ORGANIZATION_BLOCK OB 1
BEGIN
	// Check ANY pointer parameters
	CALL		FC 1 (
		FCANY1		:= P#M 10.0 BYTE 7,
		FCANY2		:= P#M 11.1 BOOL 13,
		FCANY3		:= M 12.2,
		FCANY4		:= P#DB50.DBX 10.0 DWORD 8,
		FCANY5		:= DB50.DBD 10,
		FCANY6		:= P#DBX 20.2 WORD 7,
		FCANY7		:= DB100.DBVAR2[2].V2,
		FCANY8		:= P#DB100.DBVAR2[2].V2, // awlsim extension
		FCANY9		:= P#DB100.DBVAR3, // awlsim extension
		FCANY10		:= P#DB100.DBVAR4, // awlsim extension
	)
	CALL		FB 1, DB 1 (
		FBANY1		:= P#M 10.0 BYTE 7,
		FBANY2		:= P#M 11.1 BOOL 13,
		FBANY3		:= M 12.2,
		FBANY4		:= P#DB50.DBX 10.0 DWORD 8,
		FBANY5		:= DB50.DBD 10,
		FBANY6		:= P#DBX 20.2 WORD 7,
		FBANY7		:= DB100.DBVAR2[2].V2,
		FBANY8		:= P#DB100.DBVAR2[2].V2, // awlsim extension
		FBANY9		:= P#DB100.DBVAR3, // awlsim extension
		FBANY10		:= P#DB100.DBVAR4, // awlsim extension
	)


	CALL SFC 46 // STOP CPU
END_ORGANIZATION_BLOCK


DATA_BLOCK DB 100
	STRUCT
		DBVAR1		: INT;
		DBVAR2		: ARRAY[1 .. 6] of STRUCT
			V1	: INT;
			V2	: INT;
		END_STRUCT;
		DBVAR3		: ARRAY[1 .. 4] of STRUCT
			A1	: INT;
		END_STRUCT
		DBVAR4		: ARRAY[1 .. 8] of BYTE;
	END_STRUCT;
BEGIN
END_DATA_BLOCK


FUNCTION FC 1 : VOID
	VAR_INPUT
		FCANY1		: ANY;
		FCANY2		: ANY;
		FCANY3		: ANY;
		FCANY4		: ANY;
		FCANY5		: ANY;
		FCANY6		: ANY;
		FCANY7		: ANY;
		FCANY8		: ANY;
		FCANY9		: ANY;
		FCANY10		: ANY;
	END_VAR
BEGIN
	L		P##FCANY1
	LAR1
	UD		DW#16#FF000000
	__ASSERT==	__ACCU 1,	DW#16#87000000
	L		B [AR1, P#0.0]
	__ASSERT==	__ACCU 1,	B#16#10	// S7
	L		B [AR1, P#1.0]
	__ASSERT==	__ACCU 1,	B#16#02	// BYTE
	L		W [AR1, P#2.0]
	__ASSERT==	__ACCU 1,	7	// count
	L		W [AR1, P#4.0]
	__ASSERT==	__ACCU 1,	0	// DB
	L		D [AR1, P#6.0]
	__ASSERT==	__ACCU 1,	P#M 10.0

	L		P##FCANY2
	LAR1
	UD		DW#16#FF000000
	__ASSERT==	__ACCU 1,	DW#16#87000000
	L		B [AR1, P#0.0]
	__ASSERT==	__ACCU 1,	B#16#10	// S7
	L		B [AR1, P#1.0]
	__ASSERT==	__ACCU 1,	B#16#01	// BOOL
	L		W [AR1, P#2.0]
	__ASSERT==	__ACCU 1,	13	// count
	L		W [AR1, P#4.0]
	__ASSERT==	__ACCU 1,	0	// DB
	L		D [AR1, P#6.0]
	__ASSERT==	__ACCU 1,	P#M 11.1

	L		P##FCANY3
	LAR1
	UD		DW#16#FF000000
	__ASSERT==	__ACCU 1,	DW#16#87000000
	L		B [AR1, P#0.0]
	__ASSERT==	__ACCU 1,	B#16#10	// S7
	L		B [AR1, P#1.0]
	__ASSERT==	__ACCU 1,	B#16#01	// BOOL
	L		W [AR1, P#2.0]
	__ASSERT==	__ACCU 1,	1	// count
	L		W [AR1, P#4.0]
	__ASSERT==	__ACCU 1,	0	// DB
	L		D [AR1, P#6.0]
	__ASSERT==	__ACCU 1,	P#M 12.2

	L		P##FCANY4
	LAR1
	UD		DW#16#FF000000
	__ASSERT==	__ACCU 1,	DW#16#87000000
	L		B [AR1, P#0.0]
	__ASSERT==	__ACCU 1,	B#16#10	// S7
	L		B [AR1, P#1.0]
	__ASSERT==	__ACCU 1,	B#16#06	// DWORD
	L		W [AR1, P#2.0]
	__ASSERT==	__ACCU 1,	8	// count
	L		W [AR1, P#4.0]
	__ASSERT==	__ACCU 1,	50	// DB
	L		D [AR1, P#6.0]
	__ASSERT==	__ACCU 1,	P#DBX 10.0

	L		P##FCANY5
	LAR1
	UD		DW#16#FF000000
	__ASSERT==	__ACCU 1,	DW#16#87000000
	L		B [AR1, P#0.0]
	__ASSERT==	__ACCU 1,	B#16#10	// S7
	L		B [AR1, P#1.0]
	__ASSERT==	__ACCU 1,	B#16#06	// DWORD
	L		W [AR1, P#2.0]
	__ASSERT==	__ACCU 1,	1	// count
	L		W [AR1, P#4.0]
	__ASSERT==	__ACCU 1,	50	// DB
	L		D [AR1, P#6.0]
	__ASSERT==	__ACCU 1,	P#DBX 10.0

	L		P##FCANY6
	LAR1
	UD		DW#16#FF000000
	__ASSERT==	__ACCU 1,	DW#16#87000000
	L		B [AR1, P#0.0]
	__ASSERT==	__ACCU 1,	B#16#10	// S7
	L		B [AR1, P#1.0]
	__ASSERT==	__ACCU 1,	B#16#04	// WORD
	L		W [AR1, P#2.0]
	__ASSERT==	__ACCU 1,	7	// count
	L		W [AR1, P#4.0]
	__ASSERT==	__ACCU 1,	0	// DB
	L		D [AR1, P#6.0]
	__ASSERT==	__ACCU 1,	P#DBX 20.2

	L		P##FCANY7
	LAR1
	UD		DW#16#FF000000
	__ASSERT==	__ACCU 1,	DW#16#87000000
	L		B [AR1, P#0.0]
	__ASSERT==	__ACCU 1,	B#16#10	// S7
	L		B [AR1, P#1.0]
	__ASSERT==	__ACCU 1,	B#16#05	// INT
	L		W [AR1, P#2.0]
	__ASSERT==	__ACCU 1,	1	// count
	L		W [AR1, P#4.0]
	__ASSERT==	__ACCU 1,	100	// DB
	L		D [AR1, P#6.0]
	__ASSERT==	__ACCU 1,	P#DBX 8.0

	L		P##FCANY8
	LAR1
	UD		DW#16#FF000000
	__ASSERT==	__ACCU 1,	DW#16#87000000
	L		B [AR1, P#0.0]
	__ASSERT==	__ACCU 1,	B#16#10	// S7
	L		B [AR1, P#1.0]
	__ASSERT==	__ACCU 1,	B#16#05	// INT
	L		W [AR1, P#2.0]
	__ASSERT==	__ACCU 1,	1	// count
	L		W [AR1, P#4.0]
	__ASSERT==	__ACCU 1,	100	// DB
	L		D [AR1, P#6.0]
	__ASSERT==	__ACCU 1,	P#DBX 8.0

	L		P##FCANY9
	LAR1
	UD		DW#16#FF000000
	__ASSERT==	__ACCU 1,	DW#16#87000000
	L		B [AR1, P#0.0]
	__ASSERT==	__ACCU 1,	B#16#10	// S7
	L		B [AR1, P#1.0]
	__ASSERT==	__ACCU 1,	B#16#06	// DWORD
	L		W [AR1, P#2.0]
	__ASSERT==	__ACCU 1,	2	// count
	L		W [AR1, P#4.0]
	__ASSERT==	__ACCU 1,	100	// DB
	L		D [AR1, P#6.0]
	__ASSERT==	__ACCU 1,	P#DBX 26.0

	L		P##FCANY10
	LAR1
	UD		DW#16#FF000000
	__ASSERT==	__ACCU 1,	DW#16#87000000
	L		B [AR1, P#0.0]
	__ASSERT==	__ACCU 1,	B#16#10	// S7
	L		B [AR1, P#1.0]
	__ASSERT==	__ACCU 1,	B#16#02	// BYTE
	L		W [AR1, P#2.0]
	__ASSERT==	__ACCU 1,	8	// count
	L		W [AR1, P#4.0]
	__ASSERT==	__ACCU 1,	100	// DB
	L		D [AR1, P#6.0]
	__ASSERT==	__ACCU 1,	P#DBX 34.0
END_FUNCTION


FUNCTION_BLOCK FB 1
	VAR_INPUT
		FBANY1		: ANY;
		FBANY2		: ANY;
		FBANY3		: ANY;
		FBANY4		: ANY;
		FBANY5		: ANY;
		FBANY6		: ANY;
		FBANY7		: ANY;
		FBANY8		: ANY;
		FBANY9		: ANY;
		FBANY10		: ANY;
	END_VAR
BEGIN
	L		P##FBANY1
	LAR1
	UD		DW#16#FF000000
	__ASSERT==	__ACCU 1,	DW#16#85000000
	L		B [AR1, P#0.0]
	__ASSERT==	__ACCU 1,	B#16#10	// S7
	L		B [AR1, P#1.0]
	__ASSERT==	__ACCU 1,	B#16#02	// BYTE
	L		W [AR1, P#2.0]
	__ASSERT==	__ACCU 1,	7	// count
	L		W [AR1, P#4.0]
	__ASSERT==	__ACCU 1,	0	// DB
	L		D [AR1, P#6.0]
	__ASSERT==	__ACCU 1,	P#M 10.0

	L		P##FBANY2
	LAR1
	UD		DW#16#FF000000
	__ASSERT==	__ACCU 1,	DW#16#85000000
	L		B [AR1, P#0.0]
	__ASSERT==	__ACCU 1,	B#16#10	// S7
	L		B [AR1, P#1.0]
	__ASSERT==	__ACCU 1,	B#16#01	// BOOL
	L		W [AR1, P#2.0]
	__ASSERT==	__ACCU 1,	13	// count
	L		W [AR1, P#4.0]
	__ASSERT==	__ACCU 1,	0	// DB
	L		D [AR1, P#6.0]
	__ASSERT==	__ACCU 1,	P#M 11.1

	L		P##FBANY3
	LAR1
	UD		DW#16#FF000000
	__ASSERT==	__ACCU 1,	DW#16#85000000
	L		B [AR1, P#0.0]
	__ASSERT==	__ACCU 1,	B#16#10	// S7
	L		B [AR1, P#1.0]
	__ASSERT==	__ACCU 1,	B#16#01	// BOOL
	L		W [AR1, P#2.0]
	__ASSERT==	__ACCU 1,	1	// count
	L		W [AR1, P#4.0]
	__ASSERT==	__ACCU 1,	0	// DB
	L		D [AR1, P#6.0]
	__ASSERT==	__ACCU 1,	P#M 12.2

	L		P##FBANY4
	LAR1
	UD		DW#16#FF000000
	__ASSERT==	__ACCU 1,	DW#16#85000000
	L		B [AR1, P#0.0]
	__ASSERT==	__ACCU 1,	B#16#10	// S7
	L		B [AR1, P#1.0]
	__ASSERT==	__ACCU 1,	B#16#06	// DWORD
	L		W [AR1, P#2.0]
	__ASSERT==	__ACCU 1,	8	// count
	L		W [AR1, P#4.0]
	__ASSERT==	__ACCU 1,	50	// DB
	L		D [AR1, P#6.0]
	__ASSERT==	__ACCU 1,	P#DBX 10.0

	L		P##FBANY5
	LAR1
	UD		DW#16#FF000000
	__ASSERT==	__ACCU 1,	DW#16#85000000
	L		B [AR1, P#0.0]
	__ASSERT==	__ACCU 1,	B#16#10	// S7
	L		B [AR1, P#1.0]
	__ASSERT==	__ACCU 1,	B#16#06	// DWORD
	L		W [AR1, P#2.0]
	__ASSERT==	__ACCU 1,	1	// count
	L		W [AR1, P#4.0]
	__ASSERT==	__ACCU 1,	50	// DB
	L		D [AR1, P#6.0]
	__ASSERT==	__ACCU 1,	P#DBX 10.0

	L		P##FBANY6
	LAR1
	UD		DW#16#FF000000
	__ASSERT==	__ACCU 1,	DW#16#85000000
	L		B [AR1, P#0.0]
	__ASSERT==	__ACCU 1,	B#16#10	// S7
	L		B [AR1, P#1.0]
	__ASSERT==	__ACCU 1,	B#16#04	// WORD
	L		W [AR1, P#2.0]
	__ASSERT==	__ACCU 1,	7	// count
	L		W [AR1, P#4.0]
	__ASSERT==	__ACCU 1,	0	// DB
	L		D [AR1, P#6.0]
	__ASSERT==	__ACCU 1,	P#DBX 20.2

	L		P##FBANY7
	LAR1
	UD		DW#16#FF000000
	__ASSERT==	__ACCU 1,	DW#16#85000000
	L		B [AR1, P#0.0]
	__ASSERT==	__ACCU 1,	B#16#10	// S7
	L		B [AR1, P#1.0]
	__ASSERT==	__ACCU 1,	B#16#05	// INT
	L		W [AR1, P#2.0]
	__ASSERT==	__ACCU 1,	1	// count
	L		W [AR1, P#4.0]
	__ASSERT==	__ACCU 1,	100	// DB
	L		D [AR1, P#6.0]
	__ASSERT==	__ACCU 1,	P#DBX 8.0

	L		P##FBANY8
	LAR1
	UD		DW#16#FF000000
	__ASSERT==	__ACCU 1,	DW#16#85000000
	L		B [AR1, P#0.0]
	__ASSERT==	__ACCU 1,	B#16#10	// S7
	L		B [AR1, P#1.0]
	__ASSERT==	__ACCU 1,	B#16#05	// INT
	L		W [AR1, P#2.0]
	__ASSERT==	__ACCU 1,	1	// count
	L		W [AR1, P#4.0]
	__ASSERT==	__ACCU 1,	100	// DB
	L		D [AR1, P#6.0]
	__ASSERT==	__ACCU 1,	P#DBX 8.0

	L		P##FBANY9
	LAR1
	UD		DW#16#FF000000
	__ASSERT==	__ACCU 1,	DW#16#85000000
	L		B [AR1, P#0.0]
	__ASSERT==	__ACCU 1,	B#16#10	// S7
	L		B [AR1, P#1.0]
	__ASSERT==	__ACCU 1,	B#16#06	// DWORD
	L		W [AR1, P#2.0]
	__ASSERT==	__ACCU 1,	2	// count
	L		W [AR1, P#4.0]
	__ASSERT==	__ACCU 1,	100	// DB
	L		D [AR1, P#6.0]
	__ASSERT==	__ACCU 1,	P#DBX 26.0

	L		P##FBANY10
	LAR1
	UD		DW#16#FF000000
	__ASSERT==	__ACCU 1,	DW#16#85000000
	L		B [AR1, P#0.0]
	__ASSERT==	__ACCU 1,	B#16#10	// S7
	L		B [AR1, P#1.0]
	__ASSERT==	__ACCU 1,	B#16#02	// BYTE
	L		W [AR1, P#2.0]
	__ASSERT==	__ACCU 1,	8	// count
	L		W [AR1, P#4.0]
	__ASSERT==	__ACCU 1,	100	// DB
	L		D [AR1, P#6.0]
	__ASSERT==	__ACCU 1,	P#DBX 34.0
END_FUNCTION_BLOCK


DATA_BLOCK DB 1
	FB 1
BEGIN
END_DATA_BLOCK
